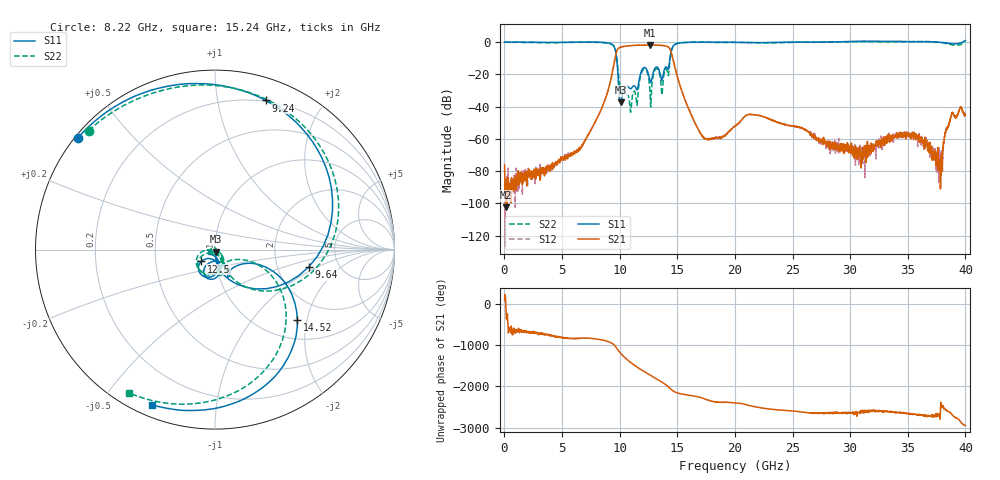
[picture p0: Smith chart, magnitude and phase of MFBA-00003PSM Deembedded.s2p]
!Keysight Technologies,N5247B,US58420632,A.15.75.19
!Date: Thursday, September 22, 2022 11:26:32
!Correction: S11(C  2-Port  )
!S41(C  2-Port  )
!S14(C  2-Port  )
!S44(C  2-Port  )
!S2P File: Measurements: S11, S41, S14, S44:
# Hz S  dB  R 50
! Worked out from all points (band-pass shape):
!   2000 points, 20 MHz to 40 GHz, reference 50 ohm
!   highest |S21| = -1.88 dB at 12.66 GHz (marker M1); lowest = -102.4 dB at 140 MHz (marker M2)
!   |S21| within 3 dB of the highest: 9.798 GHz to 14.4 GHz (4.598 GHz wide, 38 % of centre)
!   lowest |S11| = -37.4 dB at 10.1 GHz (marker M3), VSWR 1.03, Z = 50.7 - j1.15 ohm
!   |S11| at or under -10 dB: 9.739 GHz to 14.37 GHz (4.628 GHz wide, 38.4 % of centre)
!   |S22| runs from -43.5 to 0.3 dB; largest |S21 - S12| = 0.0015
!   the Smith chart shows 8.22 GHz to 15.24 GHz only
!   S11 on the Smith chart (normalised r, x): 8.22 GHz: 0.01, +0.36; 9.24 GHz: 0.19, +1.38; 9.64 GHz: 3.03, -0.81; 12.5 GHz: 0.85, -0.11; 14.52 GHz: 1.43, -1.75; 15.24 GHz: 0.05, -0.67
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2e7  -0.16 -0.5  -76.21 95.3  -88.37 151.6  -0.11 -0.5
1.4e8  -0.15 -2.8  -102.40 -131.3  -96.81 14.7  -0.11 -3.0
3.96e9  -0.26 -84.0  -76.25 -36.5  -76.43 -38.9  -0.41 -87.1
6.7e9  -0.11 -159.6  -64.63 -108.4  -64.23 -104.7  -0.17 -164.6
8.22e9  -0.13 140.8  -44.65 -139.6  -44.65 -139.6  -0.29 136.7
9.24e9  -1.13 71.2  -23.18 141.2  -23.18 141.1  -1.22 63.5
9.64e9  -5.49 -10.4  -8.71 48.5  -8.71 48.4  -5.12 -13.2
1.01e10  -37.39 -56.7  -3.18 -120.9  -3.18 -120.9  -28.63 -32.8
1.068e10  -27.41 -175.7  -2.47 84.0  -2.47 83.9  -32.66 -174.4
1.158e10  -28.13 -87.5  -2.02 -102.3  -2.03 -102.4  -33.20 -36.0
1.25e10  -19.94 -139.2  -1.91 98.8  -1.91 98.8  -21.81 -168.2
1.266e10  -24.73 -119.8  -1.88 72.4  -1.88 72.3  -34.76 -169.3
1.336e10  -16.47 -113.8  -2.05 -42.0  -2.05 -42.0  -17.53 -135.3
1.402e10  -15.42 -62.5  -2.59 -161.6  -2.59 -161.7  -16.64 -77.9
1.452e10  -4.40 -40.3  -7.60 74.9  -7.61 74.9  -4.90 -46.0
1.524e10  -0.60 -112.1  -27.08 -14.1  -27.09 -14.2  -0.62 -120.9
1.734e10  -0.08 -175.4  -59.98 -138.3  -59.64 -141.1  -0.13 -176.0
2.002e10  -0.24 124.0  -52.19 118.2  -52.10 119.5  -0.26 113.9
2.668e10  -0.17 2.8  -57.44 -129.2  -57.35 -126.7  -0.12 -4.0
3.334e10  0.40 4.7  -57.33 -96.9  -58.34 -100.2  0.06 -8.0
3.78e10  -0.16 14.7  -79.28 94.5  -70.68 25.1  -0.28 18.2
4e10  0.92 0.4  -44.83 -66.5  -44.64 -64.7  0.15 -7.9
